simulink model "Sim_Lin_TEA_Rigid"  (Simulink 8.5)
settings: Solver=ode23  StartTime=0.0  StopTime=108000  MaxStep=1  RelTol=1e-3
InitFcn:
  | start
StopFcn:
  | pl2
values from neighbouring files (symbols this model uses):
  Kpqr = lqr(sys,Q0,R0)    [des.m]
  wo = 0.0011    [start.m]    (also in start1.m; start2.m; start3.m)
undefined symbols (not defined in the file or in its folder): Av, Bv, Cv, Dv

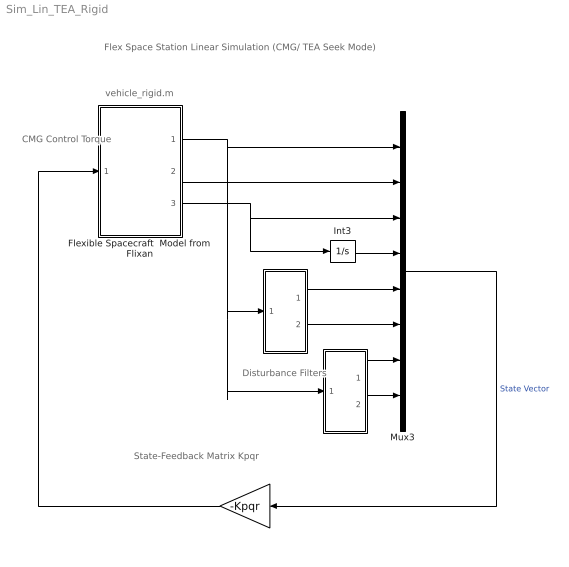
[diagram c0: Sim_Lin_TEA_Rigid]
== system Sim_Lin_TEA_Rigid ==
  note: Flex Space Station Linear Simulation (CMG/ TEA Seek Mode)
  note: State-Feedback Matrix Kpqr
  note: CMG Control Torque
  note: Disturbance Filters
  note: vehicle_rigid.m
  " " : Gain  Gain=-Kpqr  Multiplication=Matrix(K*u)
  "  " : Subsystem
  "    " : Subsystem
  Flexible Spacecraft  Model from Flixan : Subsystem
  Int3 : Integrator
  Mux3 : Mux  Inputs=[3, 3, 3, 3, 1, 1, 1, 1]
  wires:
  Int3/1 -> Mux3/4
  Mux3/1 -> " "/1  "State Vector"
  "  "/1(a1) -> Mux3/5
  "  "/2(a2) -> Mux3/6
  Flexible Spacecraft  Model from Flixan/3("Hcmg ") -> Int3/1, Mux3/3
  " "/1 -> Flexible Spacecraft  Model from Flixan/1(Tcmg)
  Flexible Spacecraft  Model from Flixan/1(att-lv) -> "    "/1(psi), "  "/1(the), Mux3/1
  Flexible Spacecraft  Model from Flixan/2(w-lv) -> Mux3/2
  "    "/1(b1) -> Mux3/7
  "    "/2(b2) -> Mux3/8

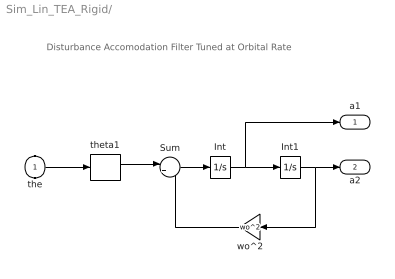
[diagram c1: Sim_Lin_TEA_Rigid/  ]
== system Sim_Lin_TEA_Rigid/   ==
  note: Disturbance Accomodation Filter Tuned at Orbital Rate
  the : Inport
  Int : Integrator
  Int1 : Integrator
  Sum : Sum  Inputs=|+-
  theta1 : Selector  InputPortWidth=3  Indices=[2]
  wo^2 : Gain  Gain=wo^2
  a1 : Outport
  a2 : Outport  Port=2
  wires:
  Int/1 -> Int1/1, a1/1
  Sum/1 -> Int/1
  Int1/1 -> wo^2/1, a2/1
  wo^2/1 -> Sum/2
  theta1/1 -> Sum/1
  the/1 -> theta1/1

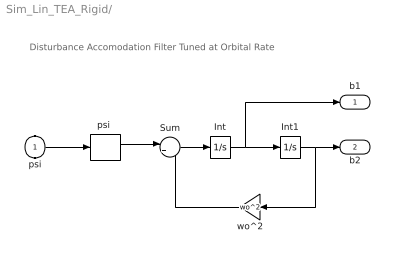
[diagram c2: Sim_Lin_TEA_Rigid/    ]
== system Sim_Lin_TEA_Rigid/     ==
  note: Disturbance Accomodation Filter Tuned at Orbital Rate
  psi : Inport
  Int : Integrator
  Int1 : Integrator
  Sum : Sum  Inputs=|+-
  "psi " : Selector  InputPortWidth=3  Indices=[3]
  wo^2 : Gain  Gain=wo^2
  b1 : Outport
  b2 : Outport  Port=2
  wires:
  Int/1 -> Int1/1, b1/1
  Sum/1 -> Int/1
  Int1/1 -> wo^2/1, b2/1
  wo^2/1 -> Sum/2
  "psi "/1 -> Sum/1
  psi/1 -> "psi "/1

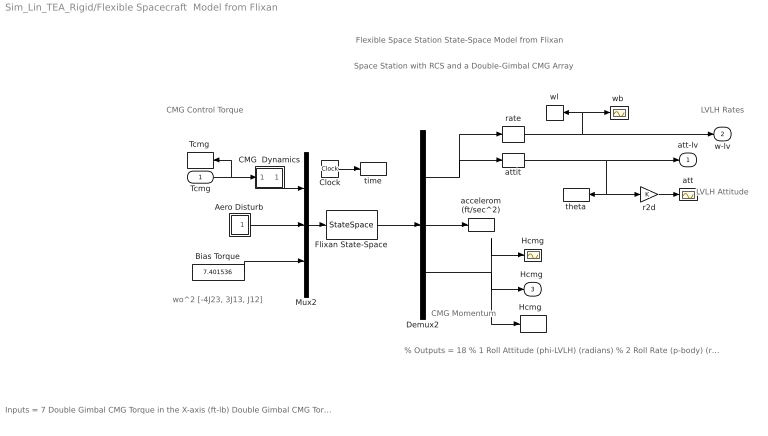
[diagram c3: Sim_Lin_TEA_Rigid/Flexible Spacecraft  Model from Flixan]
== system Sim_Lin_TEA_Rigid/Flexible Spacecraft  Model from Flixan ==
  note: Flexible Space Station State-Space Model from Flixan
  note: Space Station with RCS and a Double-Gimbal CMG Array
  note: wo^2 [-4J23, 3J13, J12]
  note: Inputs = 7 Double Gimbal CMG Torque in the X-axis (ft-lb) Double Gimbal CMG Torque in the Y-axis (ft-lb) Double Gimbal CMG Torque in the Z-axis (ft-lb) External Torque Input 1 (ft-lb), direct: External Torque Input 2 (ft-lb), direct: External Torque Input 3 (ft-lb), direct: Ext Torque Direct.=(0.197, -0.5964, -0.7782)
  note: CMG Momentum
  note: LVLH Attitude
  note: LVLH Rates
  note: CMG Control Torque
  note: % Outputs = 18 % 1 Roll Attitude (phi-LVLH) (radians) % 2 Roll Rate (p-body) (rad/sec) % 3 Pitch Attitude (thet-LVLH) (radians) % 4 Pitch Rate (q-body) (rad/sec) % 5 Yaw Attitude (psi-LVLH) (radians) % 6 Yaw Rate (r-body) (rad/sec) % 7 Angle of attack, alfa, (radians) % 8 Angle of sideslip, beta, (radian) % 9 Change in Altitude, delta-h, (feet) % 10 Forward Acceleration (V-dot) (ft/sec) % 11 Cross Range Velocity (Vcr) (ft/sec) % 12 Accelerom # 1, (along X), (ft/sec^2) Translat. Acceler % 13 Accelerom # 2, (along Z), (ft/sec^2) Translat. Acceler % 14 Accelerom # 3, (along X), (ft/sec^2) Translat. Acceler % 15 Accelerom # 4, (along Z), (ft/sec^2) Translat. Acceler % 16 Double Gimbal CMG Momentum Change in X-axis (ft-lb-sec) % 17 Double Gimbal CMG Momentum Change in Y-axis (ft-lb-sec) % 18 Double Gimbal CMG Momentum Change in Z-axis (ft-lb-sec)
  Tcmg : Inport  PortDimensions=3
  Aero Disturb : Subsystem
  Bias Torque : Constant  Value=7.401536
  CMG  Dynamics : Subsystem
  Clock : Clock
  Demux2 : Demux  Outputs=[11, 4, 3]
  Flixan State-Space : StateSpace  A=Av  B=Bv  C=Cv  D=Dv  X0=0
  Hcmg : Scope
  "Hcmg  " : ToWorkspace  VariableName=Hcmg  SampleTime=-1
  Mux2 : Mux  Inputs=[3, 3, 1]
  "Tcmg " : ToWorkspace  VariableName=Tcmg  SampleTime=-1
  accelerom (ft/sec^2) : ToWorkspace  VariableName=accel  SampleTime=-1
  att : Scope
  attit : Selector  InputPortWidth=11  Indices=[1,3,5]
  r2d : Gain
  rate : Selector  InputPortWidth=11  Indices=[2, 4, 6]
  theta : ToWorkspace  VariableName=theta  SampleTime=-1
  time : ToWorkspace  VariableName=time  SampleTime=-1
  "wb " : Scope
  wl : ToWorkspace  VariableName=wl  SampleTime=-1
  att-lv : Outport
  w-lv : Outport  Port=2
  "Hcmg " : Outport  Port=3
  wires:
  Mux2/1 -> Flixan State-Space/1
  Clock/1 -> time/1
  Demux2/3 -> "Hcmg  "/1, Hcmg/1, "Hcmg "/1
  Demux2/2 -> accelerom (ft/sec^2)/1
  attit/1 -> att-lv/1, r2d/1, theta/1
  Tcmg/1 -> CMG  Dynamics/1(I), "Tcmg "/1
  Flixan State-Space/1 -> Demux2/1
  Demux2/1 -> attit/1, rate/1
  rate/1 -> w-lv/1, wl/1, "wb "/1
  r2d/1 -> att/1
  Aero Disturb/1(Td) -> Mux2/2
  Bias Torque/1 -> Mux2/3
  CMG  Dynamics/1(O) -> Mux2/1

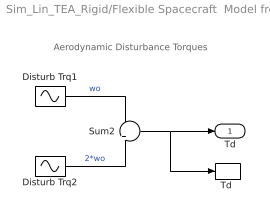
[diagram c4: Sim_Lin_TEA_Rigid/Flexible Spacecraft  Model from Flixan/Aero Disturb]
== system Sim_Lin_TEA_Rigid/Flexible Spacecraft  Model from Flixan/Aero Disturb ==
  note: Aerodynamic Disturbance Torques
  Disturb Trq1 : Sin  Amplitude=[1, 3, 1]  Bias="[1  8  1]"  Frequency=[wo, wo, wo]  SampleTime=0
  Disturb Trq2 : Sin  Amplitude=[1, 1, 1]*0.5  Frequency=[wo, wo, wo]*2  SampleTime=0
  Sum2 : Sum  Inputs=+|+
  "Td " : ToWorkspace  VariableName=Td  SampleTime=-1
  Td : Outport
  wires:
  Disturb Trq1/1 -> Sum2/1  "wo"
  Sum2/1 -> Td/1, "Td "/1
  Disturb Trq2/1 -> Sum2/2  "2*wo"

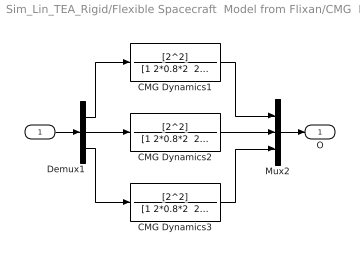
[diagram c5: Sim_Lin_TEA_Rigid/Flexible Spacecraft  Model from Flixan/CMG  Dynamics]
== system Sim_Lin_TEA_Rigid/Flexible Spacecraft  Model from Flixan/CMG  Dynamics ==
  I : Inport
  CMG Dynamics1 : TransferFcn  Numerator=[2^2]  Denominator="[1 2*0.8*2  2^2]"
  CMG Dynamics2 : TransferFcn  Numerator=[2^2]  Denominator="[1 2*0.8*2  2^2]"
  CMG Dynamics3 : TransferFcn  Numerator=[2^2]  Denominator="[1 2*0.8*2  2^2]"
  Demux1 : Demux  Outputs=3
  Mux2 : Mux  Inputs=3
  O : Outport
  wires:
  Mux2/1 -> O/1
  I/1 -> Demux1/1
  Demux1/3 -> CMG Dynamics3/1
  Demux1/1 -> CMG Dynamics1/1
  Demux1/2 -> CMG Dynamics2/1
  CMG Dynamics1/1 -> Mux2/1
  CMG Dynamics3/1 -> Mux2/3
  CMG Dynamics2/1 -> Mux2/2
